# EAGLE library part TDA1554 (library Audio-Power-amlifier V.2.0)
The TDA1554Q is an integrated class-B output amplifier in a 17-lead single-in-line (SIL) plastic power package. The circuit contains 4 x 11 W single-ended or 2 x 22 W bridge amplifiers. The device is primarily developed for car radio applications.
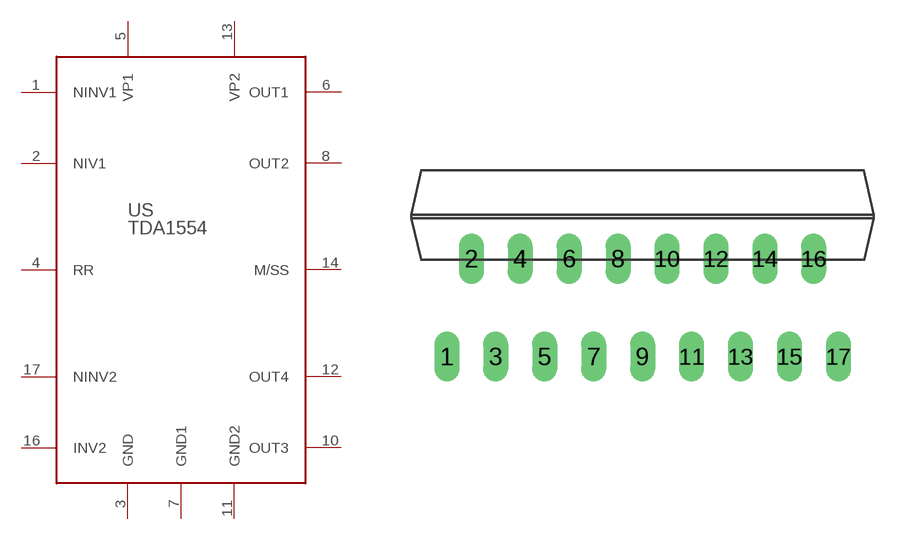
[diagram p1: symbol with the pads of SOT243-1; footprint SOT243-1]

Designator prefix US

## TDA1554Q  [SOT243-1]
1  NINV1  in
2  NIV1  in
3  GND  pwr
4  RR  pas
5  VP1  pwr
6  OUT1  out
7  GND1  pwr
8  OUT2  out
10  OUT3  out
11  GND2  pwr
12  OUT4  out
13  VP2  pwr
14  M/SS  pas
16  INV2  in
17  NINV2  in

## Footprint SOT243-1 (pad centres in mm)
DBS17P: plastic DIL-bent-SIL power package; 17 leads (lead length 7.7 mm)
drill 0.8 long: 1 -10.16,-5.08; 2 -8.89,0; 3 -7.62,-5.08; 4 -6.35,0; 5 -5.08,-5.08; 6 -3.81,0; 7 -2.54,-5.08; 8 -1.27,0; 9 0,-5.08; 10 1.27,0; 11 2.54,-5.08; 12 3.81,0; 13 5.08,-5.08; 14 6.35,0; 15 7.62,-5.08; 16 8.89,0; 17 10.17,-5.08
